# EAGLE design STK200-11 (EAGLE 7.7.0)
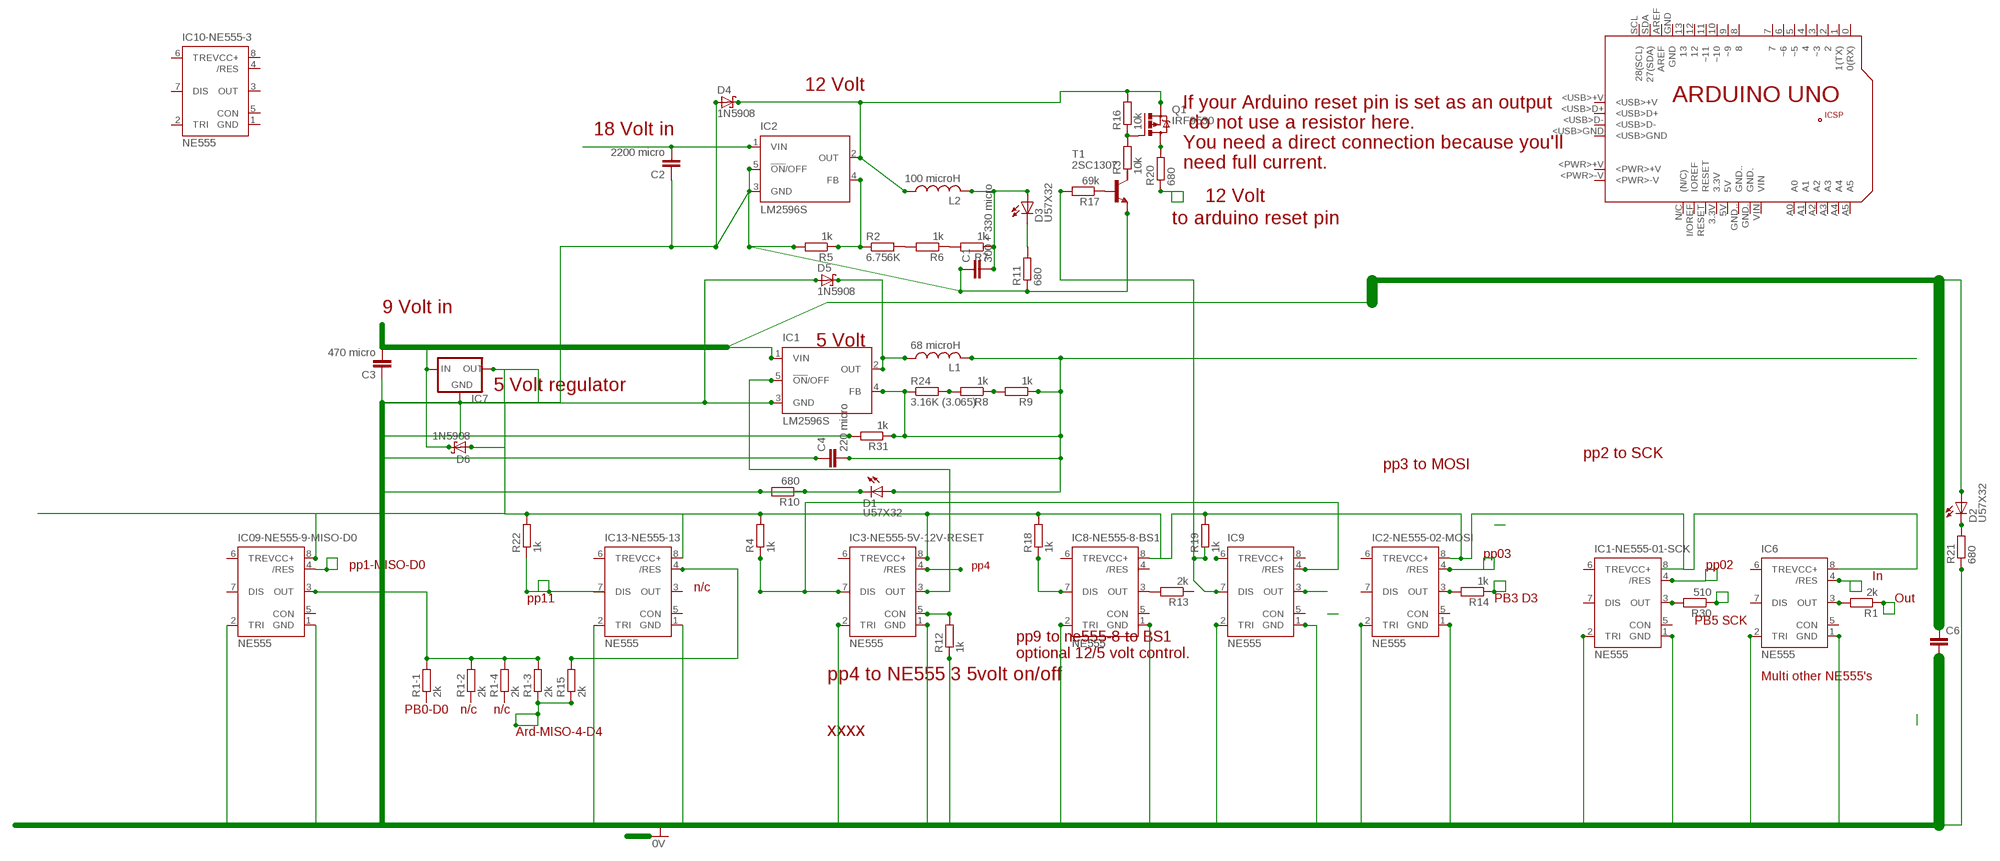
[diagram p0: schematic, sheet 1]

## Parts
C1  300 + 330 micro  C-EU050H075X075  [C050H075X075]
C2  2200 micro  C-EU050H075X075  [C050H075X075]
C3  470 micro  C-EU050H075X075  [C050H075X075]
C4  220 micro  C-EU050H075X075  [C050H075X075]
C6  C-EU050H075X075  [C050H075X075]
D1  U57X32  [U57X32]
D2  U57X32  [U57X32]
D3  U57X32  [U57X32]
D4  1N5908  [C4111-15]
D5  1N5908  [C4111-15]
D6  1N5908  [C4111-15]
IC1  LM2596S  [TO263-5]
IC1-NE555-01-SCK  NE555  [DIL-08]
IC2  LM2596S  [TO263-5]
IC2-NE555-02-MOSI  NE555  [DIL-08]
IC3-NE555-5V-12V-RESET  NE555  [DIL-08]
IC6  NE555  [DIL-08]
IC7  78XXL  [78XXL]
IC8-NE555-8-BS1  NE555  [DIL-08]
IC9  NE555  [DIL-08]
IC09-NE555-9-MISO-D0  NE555  [DIL-08]
IC10-NE555-3  NE555  [DIL-08]
IC13-NE555-13  NE555  [DIL-08]
L1  68 microH  L-US0204/5  [0204/5]
L2  100 microH  L-US0204/5  [0204/5]
PCB1  ARDUINO_UNO  [ARDUINO_UNO]
Q1  IRF9530  [TO220BV]
R1  2k  R-EU_0207/10  [0207/10]
R1-1  2k  R-EU_0207/10  [0207/10]
R1-2  2k  R-EU_0207/10  [0207/10]
R1-3  2k  R-EU_0207/10  [0207/10]
R1-4  2k  R-EU_0207/10  [0207/10]
R2  6.756K  R-EU_0207/10  [0207/10]
R3  10k  R-EU_0207/10  [0207/10]
R4  1k  R-EU_0207/10  [0207/10]
R5  1k  R-EU_0207/10  [0207/10]
R6  1k  R-EU_0207/10  [0207/10]
R7  1k  R-EU_0207/10  [0207/10]
R8  1k  R-EU_0207/10  [0207/10]
R9  1k  R-EU_0207/10  [0207/10]
R10  680  R-EU_0207/10  [0207/10]
R11  680  R-EU_0207/10  [0207/10]
R12  1k  R-EU_0207/10  [0207/10]
R13  2k  R-EU_0207/10  [0207/10]
R14  1k  R-EU_0207/10  [0207/10]
R15  2k  R-EU_0207/10  [0207/10]
R16  10k  R-EU_0207/10  [0207/10]
R17  69k  R-EU_0207/10  [0207/10]
R18  1k  R-EU_0207/10  [0207/10]
R19  1k  R-EU_0207/10  [0207/10]
R20  680  R-EU_0207/10  [0207/10]
R21  680  R-EU_0207/10  [0207/10]
R22  1k  R-EU_0207/10  [0207/10]
R24  3.16K (3.065)  R-EU_0207/10  [0207/10]
R30  510  R-EU_0207/10  [0207/10]
R31  1k  R-EU_0207/10  [0207/10]
T1  2SC1307  [TO220AV]

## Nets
+18V: D2.A
N$1: IC8-NE555-8-BS1.3(OUT) R13.2
N$2: IC9.3(OUT)
N$4: IC3-NE555-5V-12V-RESET.4(/RES)
N$5: D4.C IC2.2(OUT) L2.1 Q1.S R16.2
N$6: D2.K(C) R21.2
N$7: IC2.4(FB) R2.1 R5.1
N$8: R2.2 R6.2
N$9: C1.1 C2.1 C3.1 C4.1 C6.2 D1.K(C) D4.A D5.A IC1-NE555-01-SCK.1(GND) IC1-NE555-01-SCK.2(TRI) IC1.3(GND) IC2-NE555-02-MOSI.1(GND) IC2-NE555-02-MOSI.2(TRI) IC2.3(GND) IC2.5(!ON!/OFF) IC3-NE555-5V-12V-RESET.1(GND) IC3-NE555-5V-12V-RESET.2(TRI) IC6.1(GND) IC6.2(TRI) IC7.GND IC8-NE555-8-BS1.1(GND) IC8-NE555-8-BS1.2(TRI) IC9.1(GND) IC9.2(TRI) R5.2 R10.1 R10.2 R11.1 R12.1 R21.1 R31.2 T1.3(E)
N$10: IC3-NE555-5V-12V-RESET.5(CON) R12.2
N$11: D5.C IC1.2(OUT) L1.1
N$12: IC1.5(!ON!/OFF) IC3-NE555-5V-12V-RESET.3(OUT)
N$13: C1.2 D3.A L2.2 R7.1
N$15: IC2-NE555-02-MOSI.3(OUT) R14.2
N$17: IC1-NE555-01-SCK.3(OUT) R30.2
N$18: R6.1 R7.2
N$19: D3.K(C) R11.2
N$20: IC8-NE555-8-BS1.7(DIS) R18.1
N$21: C4.2 D1.A IC1.4(FB) L1.2 R9.1 R24.1 R31.1
N$22: C2.2 IC2.1(VIN)
N$23: R8.2 R24.2
N$24: R8.1 R9.2
N$25: Q1.G R3.2 R16.1
N$26: C3.2 D6.C IC1.1(VIN) IC7.IN
N$27: R17.1 T1.1(B)
N$28: IC9.7(DIS) R17.2 R19.1
N$31: D6.A IC2-NE555-02-MOSI.8(VCC+) IC3-NE555-5V-12V-RESET.8(VCC+) IC6.8(VCC+) IC7.OUT IC8-NE555-8-BS1.8(VCC+) IC09-NE555-9-MISO-D0.8(VCC+) R4.2 R18.2 R19.2 R22.2
N$32: IC09-NE555-9-MISO-D0.3(OUT) R1-1.2 R1-2.2 R1-3.2 R1-4.2
N$33: IC2-NE555-02-MOSI.4(/RES)
N$34: IC3-NE555-5V-12V-RESET.7(DIS) IC9.4(/RES) R4.1
N$35: IC9.6(TRE)
N$36: Q1.D R20.2
N$37: IC09-NE555-9-MISO-D0.4(/RES)
N$38: R20.1
N$39: R1-3.1 R15.1
N$40: IC13-NE555-13.4(/RES) R15.2
N$41: IC1-NE555-01-SCK.4(/RES)
N$42: R30.1
N$43: R14.1
N$44: IC6.4(/RES)
N$45: IC6.3(OUT) R1.2
N$46: R1.1
Unconnected: C6.1 IC1-NE555-01-SCK.5(CON) IC1-NE555-01-SCK.6(TRE) IC1-NE555-01-SCK.7(DIS) IC2-NE555-02-MOSI.5(CON) IC2-NE555-02-MOSI.6(TRE) IC2-NE555-02-MOSI.7(DIS) IC3-NE555-5V-12V-RESET.6(TRE) IC6.5(CON) IC6.6(TRE) IC6.7(DIS) IC8-NE555-8-BS1.4(/RES) IC8-NE555-8-BS1.5(CON) IC8-NE555-8-BS1.6(TRE) IC09-NE555-9-MISO-D0.2(TRI) IC09-NE555-9-MISO-D0.5(CON) IC09-NE555-9-MISO-D0.6(TRE) IC09-NE555-9-MISO-D0.7(DIS) IC9.5(CON) IC10-NE555-3.2(TRI) IC10-NE555-3.3(OUT) IC10-NE555-3.4(/RES) IC10-NE555-3.5(CON) IC10-NE555-3.6(TRE) IC10-NE555-3.7(DIS) IC13-NE555-13.2(TRI) IC13-NE555-13.3(OUT) IC13-NE555-13.5(CON) IC13-NE555-13.6(TRE) IC13-NE555-13.7(DIS) PCB1.0(0(RX)) PCB1.1(1(TX)) PCB1.2 PCB1.3(~3) PCB1.3.3V PCB1.4 PCB1.5(~5) PCB1.5V PCB1.6(~6) PCB1.7 PCB1.8 PCB1.9(~9) PCB1.10(~10) PCB1.11(~11) PCB1.12 PCB1.13 PCB1.+5V PCB1.<PWR>+V PCB1.<PWR>-V PCB1.<USB>+V PCB1.<USB>D+ PCB1.<USB>D- PCB1.<USB>GND PCB1.A0 PCB1.A1 PCB1.A2 PCB1.A3 PCB1.A4 PCB1.A5 PCB1.AREF PCB1.GND PCB1.GND. PCB1.GND.. PCB1.GND_ PCB1.I/OREF(IOREF) PCB1.MISO PCB1.MOSI PCB1.N/C((N/C)) PCB1.RESET PCB1.RESET. PCB1.SCK PCB1.SCL(28(SCL)) PCB1.SDA(27(SDA)) PCB1.VIN R1-1.1 R1-2.1 R1-4.1 R3.1 R13.1 R22.1 T1.2(C)

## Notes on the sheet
- 12 Volt
- 18 Volt in
- If your Arduino reset pin is set as an output
   do not use a resistor here.
  You need a direct connection because you'll 
  need full current.
- 12 Volt
- to arduino reset pin
- 9 Volt in
- 5 Volt
- 5 Volt regulator
- pp2 to SCK
- pp3 to MOSI
- pp03
- pp1-MISO-D0 | pp4 | pp02
- In
- n/c
- pp11 | PB3 D3 | Out
- PB5 SCK
- pp9 to ne555-8 to BS1
  optional 12/5 volt control.
- pp4 to NE555 3 5volt on/off | Multi other NE555's
- PB0-D0 | n/c | n/c
- Ard-MISO-4-D4 | xxxx

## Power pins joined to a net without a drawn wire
GND: IC09-NE555-9-MISO-D0.1(GND) IC10-NE555-3.1(GND) IC13-NE555-13.1(GND)
VCC+: IC1-NE555-01-SCK.8(VCC+) IC9.8(VCC+) IC10-NE555-3.8(VCC+) IC13-NE555-13.8(VCC+)

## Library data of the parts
C1-C4 C6 = rcl:C-EU: CAPACITOR, European symbol
D1-D3 = led:U57X32: LED
D4-D6 = diode:1N5908: DIODE
IC1 IC2 = national-semiconductor:LM2596: SIMPLE SWITCHER® Power Converter 150 kHz 3A Step-Down Voltage Regulator Source: http://www.national.com/ds/LM/LM2596.pdf; MF: NATIONAL SEMICONDUCTOR; MPN: LM2596S-ADJ/NOPB; OC_FARNELL: 9494367; OC_NEWARK: 41K3842
IC1-NE555-01-SCK IC2-NE555-02-MOSI IC3-NE555-5V-12V-RESET IC6 IC8-NE555-8-BS1 IC9 IC09-NE555-9-MISO-D0 IC10-NE555-3 IC13-NE555-13 = st-microelectronics:NE555: General purpose bipolar Timer; MF: Arrow Electronics; MPN: NE555N; OC_FARNELL: 1467742; OC_NEWARK: 89K1486
IC7 = v-reg:78XXL: VOLTAGE REGULATOR
L1 L2 = resistor:L-US: INDUCTOR, American symbol
PCB1 = E14_Arduino_revC:ARDUINO_UNO: Device for representing an Arduino Uno board with a footprint in an EAGLE design. Created by Dave Young for Element14. More EAGLE documentation at: http://www.element14.com/community/community/knode/cadsoft_eagle
Q1 = transistor-power:IRF9530: P-CHANNEL HEXFET POWER-MOS-FET Source: http://www.irf.com/product-info/datasheets/data/irf9530.pdf
R1 R1-1-R1-4 R2-R22 R24 R30 R31 = rcl:R-EU_: RESISTOR, European symbol
T1 = transistor-neu-to92:2SC1307: NPN Transistor Silicon Epitaxial, High Frequency Power Amplifier Source: 2SC1307.pdf

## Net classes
0 default: clearance 0.205 mm

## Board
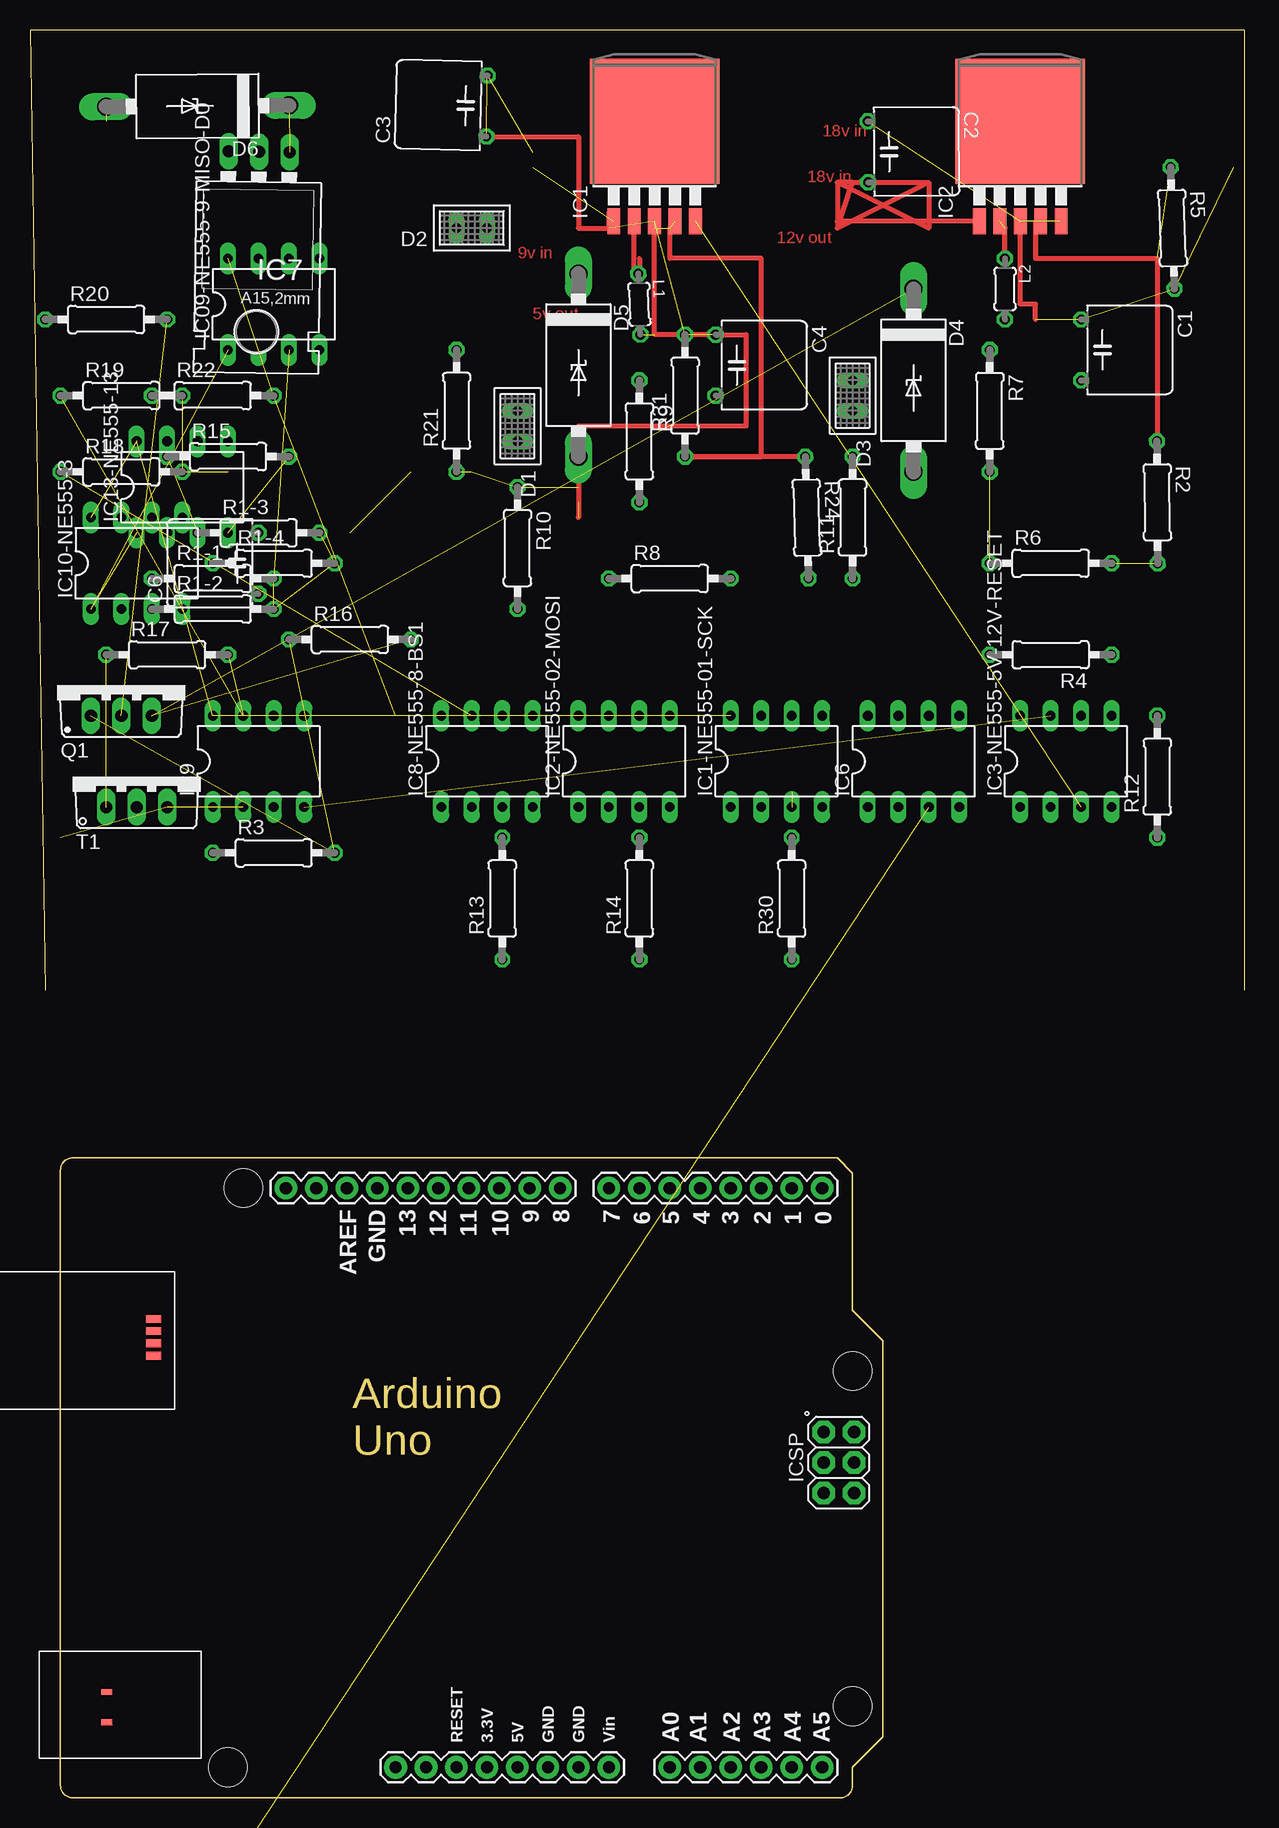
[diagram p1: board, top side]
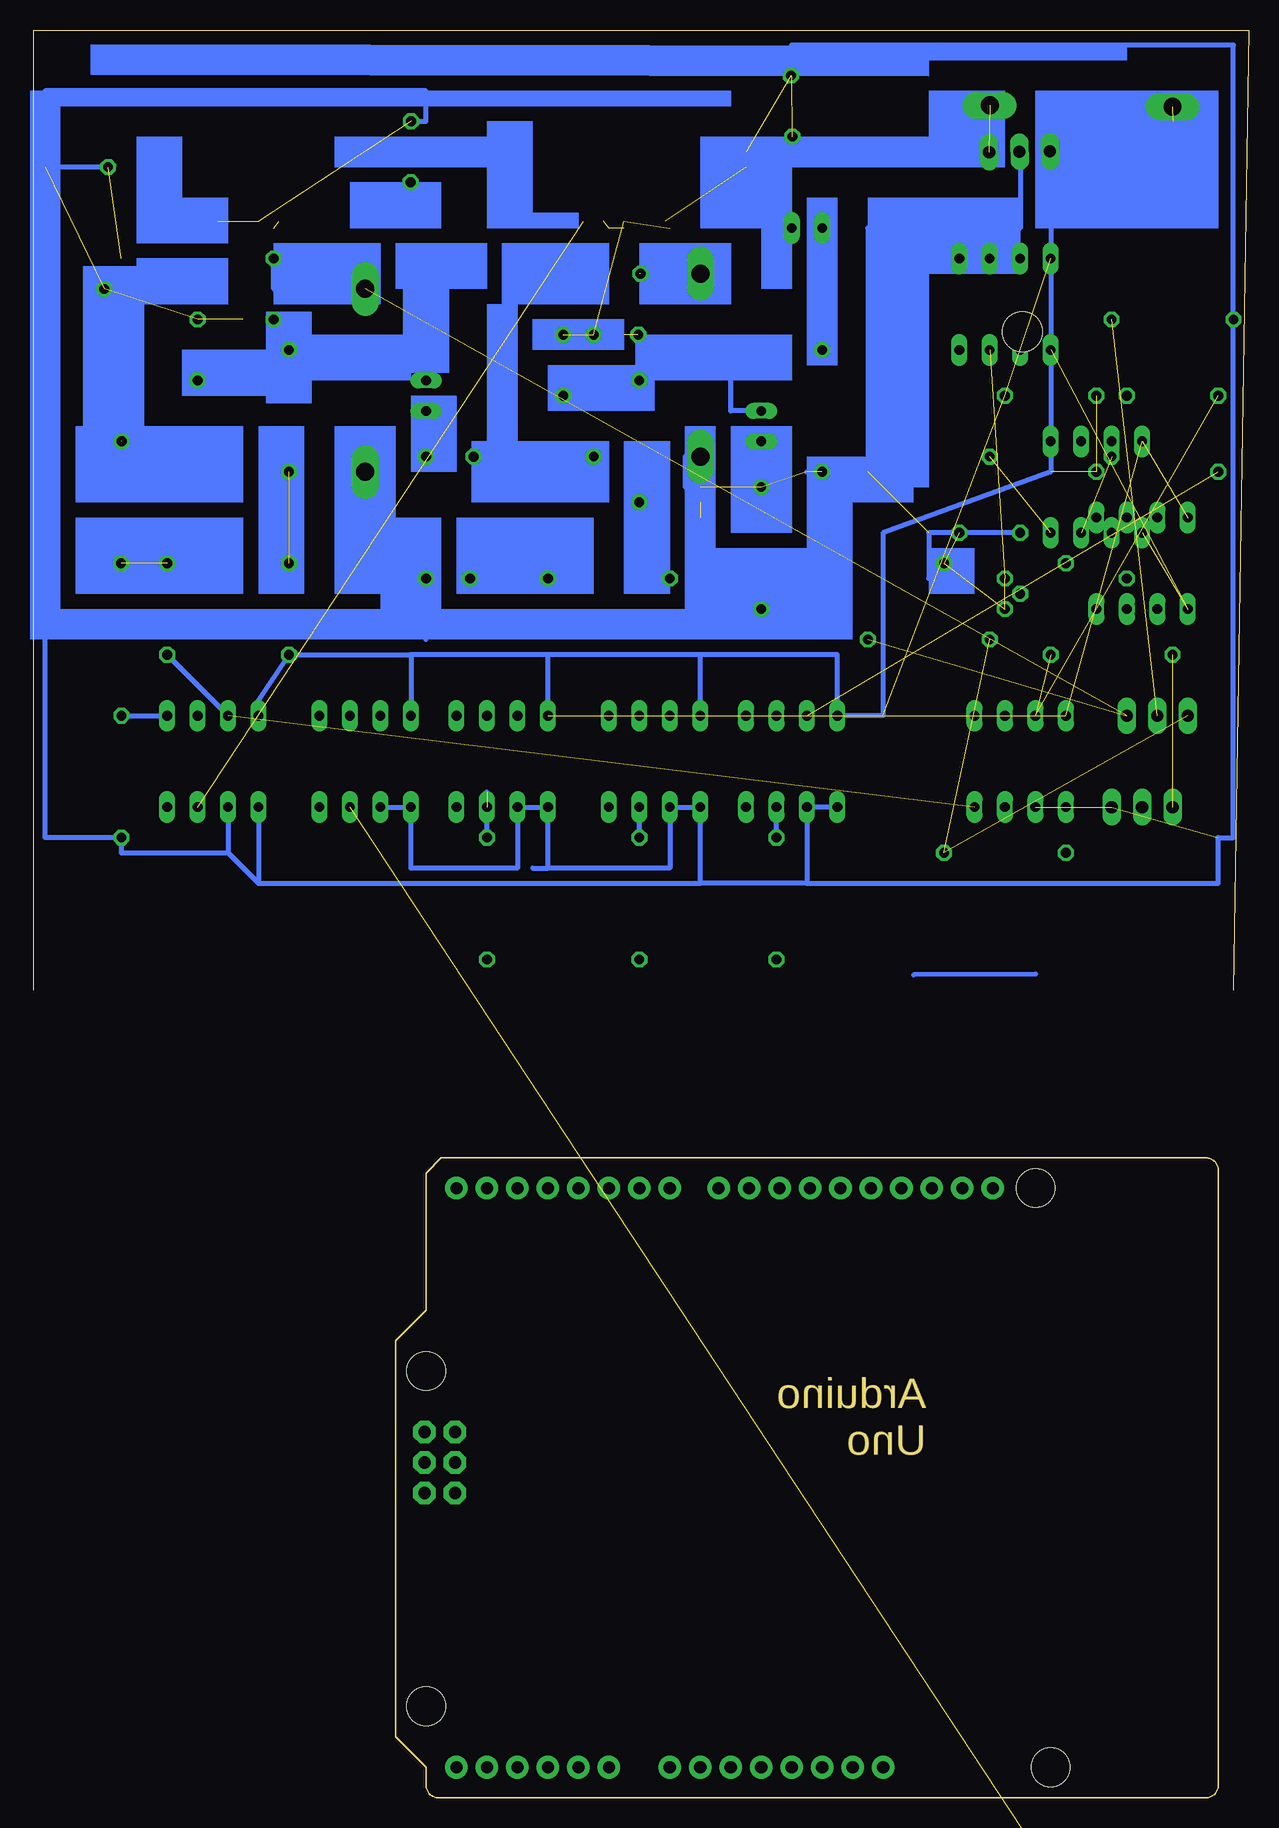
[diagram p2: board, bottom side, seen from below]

Size 101.27 x 147.31 mm. Coordinates in mm from the lower left corner, seen from the top.
Outline: 101.27,67.31 101.27,147.31 0,147.31 1.27,67.31
Copper layers (1*16): Top 0.035mm / dielectric 1.5mm / Bottom 0.035mm
Design rules "default": minimum track width 10mil, minimum drill 24mil, track to track 8mil, track to pad 8mil, pad to pad 8mil, via to via 8mil, smd to smd 8mil, copper to edge 40mil, drill to drill 8mil, minimum pad ring 10mil, minimum via ring 8mil, stop-mask expansion 4mil, vias tented up to drill 0mil, thermal gap 10mil

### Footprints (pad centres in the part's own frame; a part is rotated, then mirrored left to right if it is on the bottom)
C050H075X075 = drill 0.813 octagon: 1 -2.54,0; 2 2.54,0
U57X32 = drill 0.813 long: A -1.27,0; K 1.27,0
C4111-15 = drill 1.499 long: A 7.62,0; C -7.62,0
TO263-5 = smd 1.067 x 2.159: 1 -3.404,-5.791; 2 -1.702,-5.791; 3 0,-5.791; 4 1.702,-5.791; 5 3.404,-5.791 | smd 10.8 x 10.41: 6 0,2.54
DIL-08 = drill 0.813 long: 1 -3.81,-3.81; 2 -1.27,-3.81; 3 1.27,-3.81; 4 3.81,-3.81; 5 3.81,3.81; 6 1.27,3.81; 7 -1.27,3.81; 8 -3.81,3.81
78XXL = drill 1.016 long: GND 0,-3.81; IN -2.54,-3.81; OUT 2.54,-3.81 | hole 3.302: 0,11.176
0204/5 = drill 0.813 octagon: 1 -2.54,0; 2 2.54,0
ARDUINO_UNO = drill 1.016 pad 1.88: 0 63.5,50.8; 1 60.96,50.8; 2 58.42,50.8; 3 55.88,50.8; 3.3V 35.56,2.54; 4 53.34,50.8; 5 50.8,50.8; 5V 38.1,2.54; 6 48.26,50.8; 7 45.72,50.8; 8 41.656,50.8; 9 39.116,50.8; 10 36.576,50.8; 11 34.036,50.8; 12 31.496,50.8; 13 28.956,50.8; A0 50.8,2.54; A1 53.34,2.54; A2 55.88,2.54; A3 58.42,2.54; A4 60.96,2.54; A5 63.5,2.54; AREF 23.876,50.8; GND 26.416,50.8; GND. 43.18,2.54; GND.. 40.64,2.54; I/OREF 30.48,2.54; N/C 27.94,2.54; RESET 33.02,2.54; SCL 18.796,50.8; SDA 21.336,50.8; VIN 45.72,2.54 | drill 1.016 pad 1.88 octagon: +5V 66.167,30.48; GND_ 66.167,25.4; MISO 63.627,30.48; MOSI 66.167,27.94; RESET. 63.627,25.4; SCK 63.627,27.94 | smd 1.016 x 0.508: <PWR>+V 3.861,8.814; <PWR>-V 3.861,6.274 | smd 1.27 x 0.635: <USB>+V 7.772,39.878; <USB>D+ 7.772,38.887; <USB>D- 7.772,37.871; <USB>GND 7.772,36.83 | hole 3.2: 66.04,7.62; 66.04,35.56; 15.24,50.8; 13.97,2.54
TO220BV = drill 1.016 long: D 0,-2.54; G -2.54,-2.54; S 2.54,-2.54
0207/10 = drill 0.813 octagon: 1 -5.08,0; 2 5.08,0
TO220AV = drill 1.016 long: 1 -2.54,-2.54; 2 0,-2.54; 3 2.54,-2.54

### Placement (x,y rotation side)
C1  87.63,120.65 270 top
C2  69.85,137.16 270.4 top
C3  38.1,140.97 88.7 top
C4  57.15,119.38 270 top
C6  19.05,102.87 90 top
D1  40.64,114.3 270 top
D2  36.83,130.81 180 top
D3  68.58,116.84 270 top
D4  73.66,118.11 270 top
D5  45.72,119.38 270 top
D6  13.97,140.97 180.4 top
IC1  52.07,137.16 0 top
IC1-NE555-01-SCK  62.23,86.36 0 top
IC2  82.55,137.16 0 top
IC2-NE555-02-MOSI  49.53,86.36 0 top
IC3-NE555-5V-12V-RESET  86.36,86.36 0 top
IC6  73.66,86.36 0 top
IC7  19.05,133.35 179.1 top
IC8-NE555-8-BS1  38.1,86.36 0 top
IC9  19.05,86.36 0 top
IC09-NE555-9-MISO-D0  20.32,124.46 0 top
IC10-NE555-3  8.89,102.87 0 top
IC13-NE555-13  12.7,109.22 0 top
L1  50.8,124.46 272.1 top
L2  81.28,125.73 270 top
PCB1  2.54,0 0 top
Q1  7.62,92.71 0 top
R1  not placed on the board
R1-1  15.24,101.6 0 top
R1-2  15.24,99.06 0 top
R1-3  19.05,105.41 0 top
R1-4  20.32,102.87 0 top
R2  93.98,107.95 270.3 top
R3  20.32,78.74 0 top
R4  85.09,95.25 180 top
R5  95.25,130.81 271.8 top
R6  85.09,102.87 0 top
R7  80.01,115.57 270 top
R8  53.34,101.6 0 top
R9  50.8,113.03 270 top
R10  40.64,104.14 270 top
R11  68.58,106.68 90 top
R12  93.98,85.09 90 top
R13  39.37,74.93 90 top
R14  50.8,74.93 90 top
R15  16.51,111.76 0 top
R16  26.67,96.52 0 top
R17  11.43,95.25 0 top
R18  7.62,110.49 0 top
R19  7.62,116.84 0 top
R20  6.35,123.19 0 top
R21  35.56,115.57 90 top
R22  15.24,116.84 0 top
R24  64.77,106.68 271.6 top
R30  63.5,74.93 90 top
R31  54.61,116.84 90 top
T1  8.89,85.09 0 top

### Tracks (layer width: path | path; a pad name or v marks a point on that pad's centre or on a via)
+18V
  Top 0.406: 38.1,131.37 D2.A
GND  (2 unrouted)
N$1
  Bottom 0.406: R13.2 IC8-NE555-8-BS1.3
N$3
  Bottom 0.406: 69.85,139.7 68.58,139.7 68.58,142.24 100.33,142.24 100.33,97.79 68.58,97.79 68.58,96.52
N$5  (3 unrouted)
  Top 0.406: L2.1 81.28,130.81
  Bottom 0.406: D4.C 81.28,125.73 L2.1
N$6
  Bottom 0.406: R21.2 D2.K
N$7  (2 unrouted)
  Top 0.406: IC2.4 83.82,131.37 83.82,128.27 93.98,128.27 93.98,113.03
  Bottom 0.406: R5.1 100.33,135.89 | 100.33,135.89 | 100.33,135.89 100.33,134.62
N$8  (1 unrouted)
N$9  (18 unrouted)
  Top 0.406: C3.1 45.72,138.43 45.72,130.81 48.26,130.81 48.26,132.08 | 83.82,123.19 83.82,124.46 82.55,124.46 IC2.3 | C4.1 59.69,121.92 59.69,114.3 45.72,114.3 45.72,106.68
  Bottom 0.406: 67.9,98.67 67.31,97.79 45.72,97.79 45.72,99.06 | 67.9,98.67 72.39,105.41 72.39,110.49 D4.A | 45.72,99.06 45.72,106.68 | R10.1 D1.K | 45.72,99.06 R10.2 40.64,97.79 35.56,97.79 | R11.1 67.9,101.6 67.9,98.67 | IC7.GND 19.05,137.16 19.05,130.81 31.75,130.81 31.75,110.49 36.83,110.49 | D5.A 46.99,111.76 46.99,109.22 45.72,109.22 45.72,107.95 | 26.67,101.6 26.67,105.41 C6.2 | IC8-NE555-8-BS1.1 IC8-NE555-8-BS1.2 36.83,76.2 | 36.83,76.2 45.72,76.2 | 45.72,76.2 IC2-NE555-02-MOSI.1 IC2-NE555-02-MOSI.2 48.26,77.47 58.42,77.47 | 59.69,77.47 58.42,77.47 | 58.42,77.47 IC1-NE555-01-SCK.1 IC1-NE555-01-SCK.2 60.96,77.47 69.85,77.47 IC6.1 IC6.2 | 85.09,78.74 93.98,78.74 R12.1 100.33,80.01 100.33,135.89 | 85.09,78.74 82.55,76.2 | 82.55,76.2 45.72,76.2 | IC3-NE555-5V-12V-RESET.2 85.09,78.74 | IC3-NE555-5V-12V-RESET.1 82.55,76.2 | 36.83,76.2 2.54,76.2 2.54,80.01 1.27,80.01 1.27,146.05 38.1,146.05 38.1,143.51
N$10
  Bottom 0.406: R12.2 IC3-NE555-5V-12V-RESET.5
N$11  (1 unrouted)
  Top 0.406: 50.8,128.27 50.8,127 50.37,127 IC1.2
  Bottom 0.406: D5.C L1.1
N$12  (1 unrouted)
N$13
  Bottom 0.406: C1.2 81.28,118.11 L2.2 81.28,120.65 R7.1 68.58,120.65 D3.A
N$15
  Bottom 0.406: R14.2 IC2-NE555-02-MOSI.3
N$16
  Bottom 0.406: 17.78,68.63 27.94,68.58
N$17  (1 unrouted)
  Bottom 0.406: R30.2 63.5,83.82
N$18  (1 unrouted)
N$19
  Bottom 0.406: D3.K R11.2
N$20  (1 unrouted)
N$21  (3 unrouted)
  Top 0.406: 57.15,121.92 52.07,121.92 52.07,130.81 | R24.1 R31.1 60.96,111.76 60.96,128.27 53.34,128.27 53.34,130.81 | L1.2
  Bottom 0.406: R9.1 50.8,119.38 50.89,119.38 L1.2 | C4.2 50.8,116.84 R9.1 | D1.A 43.18,115.57 43.18,119.38 R9.1
N$22  (1 unrouted)
  Top 0.406: IC2.1 67.31,131.37 | 67.31,130.81 68.58,134.62 | 68.58,134.62 67.31,134.62 | 67.31,134.62 67.31,131.37 | 67.31,131.37 67.31,130.81 | 74.93,134.62 67.31,130.81 | 68.58,134.62 74.93,134.62 | 74.93,134.62 74.93,130.81 67.31,134.62
  Bottom 0.406: C2.2 69.85,134.62 69.85,133.35
N$23
  Bottom 0.406: R24.2 R8.2
N$24
  Bottom 0.406: R8.1 R9.2
N$25  (2 unrouted)
N$26  (3 unrouted)
  Bottom 0.406: IC7.IN 41.91,137.12 41.91,135.89
N$27  (1 unrouted)
N$28  (2 unrouted)
N$30
  Bottom 0.406: 21.59,140.97 21.59,135.89
N$31  (5 unrouted)
  Bottom 0.406: 7.62,139.7 6.35,139.7 6.35,135.89 16.51,135.89 | IC7.OUT 16.51,137.2 16.51,135.89 | 16.51,135.89 16.51,110.49 30.48,105.41 30.48,90.17 IC8-NE555-8-BS1.8 34.29,95.25 45.72,95.25 | IC2-NE555-02-MOSI.8 45.72,95.25 | 45.72,95.25 58.42,95.25 | 58.42,90.17 58.42,95.25 | 58.42,95.25 69.85,95.25 | 69.85,95.25 IC6.8 | IC3-NE555-5V-12V-RESET.8 82.55,91.44 R4.2 69.85,95.25
N$32  (4 unrouted)
N$34  (1 unrouted)
  Bottom 0.406: IC3-NE555-5V-12V-RESET.7 R4.1
N$36  (1 unrouted)
N$39  (1 unrouted)
N$40  (1 unrouted)
N$45  (1 unrouted)
VCC+  (3 unrouted)
(copper drawn outside any net)
  shapes: Bottom area x57

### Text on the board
Top: 18v in | 18v in | 12v out | 9v in | 5v out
